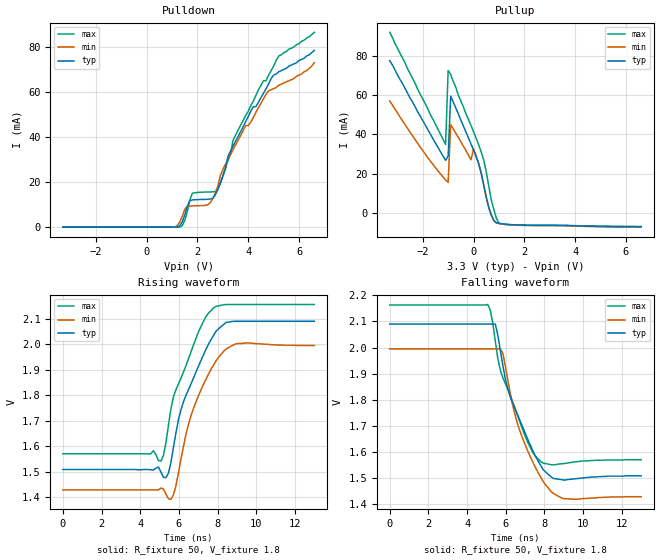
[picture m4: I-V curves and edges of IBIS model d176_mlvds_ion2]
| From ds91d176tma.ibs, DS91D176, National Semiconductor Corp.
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[Model]   d176_mlvds_ion2
Model_type I/O
Polarity Inverting
Vinh=0.05
Vinl=-0.05
Vref=1.8
Vmeas=1.8
Rref=50
Cref=0p
|   Typ   Min   Max
C_comp   9.5pF   9.5pF   9.5pF
[Model Spec]
S_overshoot_high   3.8   3.8   3.8
S_overshoot_low   -1.4   -1.4   -1.4
[Temperature Range]   25   85   -40
[Voltage Range]   3.3   3.0   3.6
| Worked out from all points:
|   slope of the pullup table from 0 to 0.495 V, typ, clamps not added: 20.8 ohm
|   rising waveform, R_fixture 50, V_fixture 1.8: 20-80 % time 1.58ns typ, 1.44ns min, 1.49ns max; typ from 1.51 V to 2.09 V
|   falling waveform, R_fixture 50, V_fixture 1.8: 20-80 % time 1.52ns typ, 1.44ns min, 1.44ns max; typ from 2.09 V to 1.51 V
[GND Clamp]
|V(groundclamp)   I(typ)   I(min)   I(max)
-3.3V     0A         0A         0A
3.3V      0A         0A         0A
[POWER Clamp]
|V(powerclamp)   I(typ)   I(min)   I(max)
-3.3V     0A         0A         0A
0V        0A         0A         0A
[Pullup]
|Vtable   I(typ)   I(min)   I(max)
-3.3V     77.5mA     57mA       92mA
-1.1V     26.7mA     16.7mA     34.8mA
-1V       28.9mA     15.5mA     72.5mA
-900mV    59.5mA     44.9mA     70.5mA
-100mV    35.1mA     27mA       44.5mA
0V        32mA       32.6mA     41.3mA
200mV     24.9mA     25.4mA     34.7mA
400mV     14mA       14.3mA     26.9mA
700mV     -1.18mA    -1.2mA     6.45mA
900mV     -5.1mA     -5.2mA     -2.87mA
1V        -5.4mA     -5.5mA     -5.25mA
6.6V      -7.2mA     -7.35mA    -7mA
[Pulldown]
|V(pulldown)   I(typ)   I(min)   I(max)
-3.3V     -14pA      -73pA      -14.1pA
1.1V      6.4uA      111uA      70nA
1.4V      2.31mA     4.79mA     640uA
1.7V      11.8mA     9.35mA     12mA
1.8V      12.1mA     9.45mA     15.1mA
2.4V      12.4mA     9.9mA      15.6mA
2.8V      16.6mA     18.1mA     16.8mA
3.3V      33.7mA     32.2mA     32.4mA
3.4V      36mA       34.4mA     38.5mA
4.7V      61.5mA     59mA       65mA
5.2V      69mA       63mA       76mA
6.6V      78.5mA     73mA       86.5mA
[Rising Waveform]
R_fixture=50
V_fixture=1.8
V_fixture_min=1.72
V_fixture_max=1.86
0s        1.508V     1.428V     1.57V
4.68ns    1.506V     1.428V     1.582V
5.07ns    1.498V     1.435V     1.541V
5.33ns    1.476V     1.411V     1.613V
5.59ns    1.537V     1.391V     1.748V
6.24ns    1.775V     1.601V     1.892V
6.63ns    1.845V     1.721V     1.971V
7.41ns    1.982V     1.864V     2.11V
8.32ns    2.078V     1.973V     2.155V
13ns      2.09V      1.995V     2.156V
[Falling Waveform]
R_fixture=50
V_fixture=1.8
V_fixture_min=1.72
V_fixture_max=1.86
0s        2.09V      1.995V     2.163V
5.07ns    2.09V      1.995V     2.165V
5.46ns    2.09V      1.995V     2.024V
5.72ns    1.988V     1.995V     1.912V
6.11ns    1.841V     1.873V     1.839V
6.76ns    1.716V     1.674V     1.708V
7.41ns    1.602V     1.559V     1.596V
8.32ns    1.506V     1.45V      1.551V
9.49ns    1.496V     1.418V     1.561V
13ns      1.508V     1.428V     1.57V
[Ramp]
|   typ   min   max
dV/dt_r   340m/1054p   340m/1350p   340m/806p
dV/dt_f   340m/1054p   340m/1350p   340m/806p
R_load=50
|[End   ds91d176_mlvds_io2
